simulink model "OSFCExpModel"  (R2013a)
settings: Solver=ode3  StartTime=0.0  StopTime=10  FixedStep=Ts  RelTol=1e-3
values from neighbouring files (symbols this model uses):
  k1 = K(1)    [OSFC_Constants.m]
  k2 = K(2)    [OSFC_Constants.m]
  k3 = K(3)    [OSFC_Constants.m]
  k4 = K(4)    [OSFC_Constants.m]
  Rd = 0    [OSFC_Constants.m]
  Ri = 10    [OSFC_Constants.m]
  Ts = 0.01    [OSFC_Constants.m]
libraries: arduinolib x3, THLlib x2, simulink x2

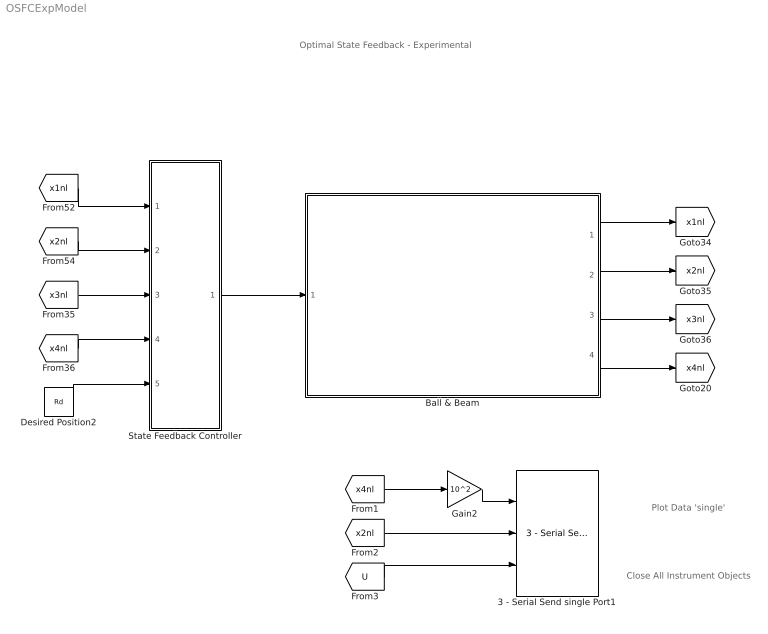
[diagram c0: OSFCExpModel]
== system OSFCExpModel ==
  note: Plot Data 'single'
  note: Close All Instrument Objects
  note: Optimal State Feedback - Experimental
  3 - Serial Send single Port1 : THLlib/3 - Serial Send  single Port0
  Ball & Beam : Subsystem
  Desired Position2 : Constant  Value=Rd
  Gain2 : Gain  Gain=10^2  SampleTime=Ts
  State Feedback Controller : Subsystem
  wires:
  [x1nl] -> State Feedback Controller/1(x1)
  [x2nl] -> State Feedback Controller/2(x2)
  [x3nl] -> State Feedback Controller/3(x3)
  [x4nl] -> State Feedback Controller/4(x4)
  Desired Position2/1 -> State Feedback Controller/5(R (desired))
  State Feedback Controller/1(U) -> Ball & Beam/1("U ")
  Ball & Beam/1(x1) -> [x1nl]
  Ball & Beam/2(x2) -> [x2nl]
  Ball & Beam/3(x3) -> [x3nl]
  Ball & Beam/4(x4) -> [x4nl]
  [x4nl] -> Gain2/1
  Gain2/1 -> 3 - Serial Send single Port1/1
  [x2nl] -> 3 - Serial Send single Port1/2
  [U] -> 3 - Serial Send single Port1/3

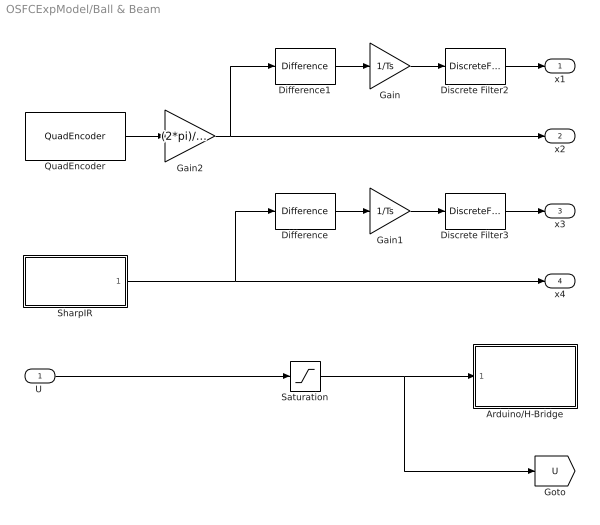
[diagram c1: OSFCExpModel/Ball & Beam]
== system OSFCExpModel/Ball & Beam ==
  "U " : Inport
  Arduino/H-Bridge : Subsystem
  Difference : simulink/Discrete/Difference  ICPrevInput=0.0  InputProcessing=Inherited  OutMin=[]  OutMax=[]  OutDataType=fixdt(1, 16)  OutScaling=2^-10  DoSatur=off
  Difference1 : simulink/Discrete/Difference  ICPrevInput=0.0  InputProcessing=Inherited  OutMin=[]  OutMax=[]  OutDataType=fixdt(1, 16)  OutScaling=2^-10  DoSatur=off
  Discrete Filter2 : DiscreteFilter  Numerator=[.4]  Denominator=[1 -0.6]  SampleTime=Ts
  Discrete Filter3 : DiscreteFilter  Numerator=[.4]  Denominator=[1 -0.6]  SampleTime=Ts
  Gain : Gain  Gain=1/Ts  SampleTime=Ts
  Gain1 : Gain  Gain=1/Ts  SampleTime=Ts
  Gain2 : Gain  Gain=(2*pi)/1336  SampleTime=Ts
  QuadEncoder : THLlib/QuadEncoder
  Saturation : Saturate  UpperLimit=12  LowerLimit=-12  SampleTime=Ts
  SharpIR : Subsystem
  x1 : Outport
  x2 : Outport  Port=2
  x3 : Outport  Port=3
  x4 : Outport  Port=4
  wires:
  "U "/1 -> Saturation/1
  Saturation/1 -> [U], Arduino/H-Bridge/1(ControlInput)
  Gain/1 -> Discrete Filter2/1
  Gain1/1 -> Discrete Filter3/1
  Difference1/1 -> Gain/1
  Difference/1 -> Gain1/1
  Discrete Filter3/1 -> x3/1
  Discrete Filter2/1 -> x1/1
  SharpIR/1(Out1) -> Difference/1, x4/1
  QuadEncoder/1 -> Gain2/1
  Gain2/1 -> x2/1, Difference1/1

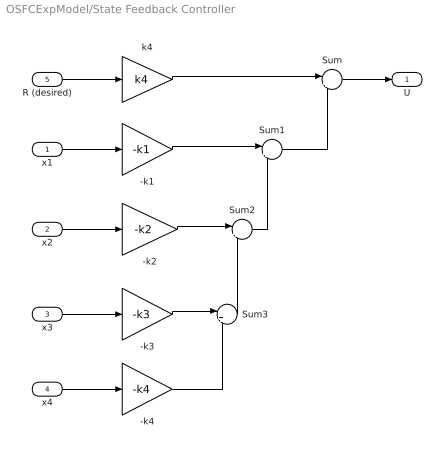
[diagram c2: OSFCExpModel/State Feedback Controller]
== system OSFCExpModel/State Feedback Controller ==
  x1 : Inport
  x2 : Inport  Port=2
  x3 : Inport  Port=3
  x4 : Inport  Port=4
  R (desired) : Inport  Port=5
  -k1 : Gain  Gain=-k1
  -k2 : Gain  Gain=-k2
  -k3 : Gain  Gain=-k3
  -k4 : Gain  Gain=-k4
  Sum{,1..3} (4 alike) : Sum  Inputs=|++
  k4 : Gain  Gain=k4
  U : Outport
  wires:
  -k4/1 -> Sum3/2
  Sum3/1 -> Sum2/2
  Sum2/1 -> Sum1/2
  Sum1/1 -> Sum/2
  Sum/1 -> U/1
  -k3/1 -> Sum3/1
  -k2/1 -> Sum2/1
  -k1/1 -> Sum1/1
  k4/1 -> Sum/1
  x4/1 -> -k4/1
  x3/1 -> -k3/1
  x2/1 -> -k2/1
  x1/1 -> -k1/1
  R (desired)/1 -> k4/1

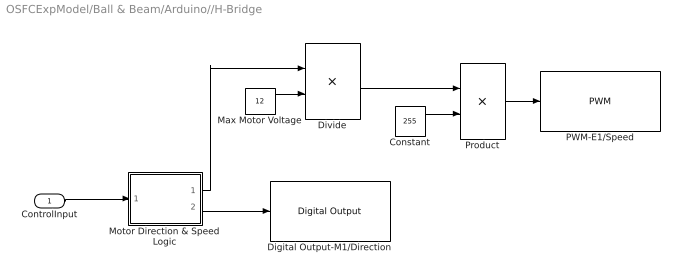
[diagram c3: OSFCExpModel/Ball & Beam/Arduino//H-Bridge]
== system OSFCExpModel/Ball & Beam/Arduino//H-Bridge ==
  ControlInput : Inport
  Constant : Constant  Value=255
  Digital Output-M1/Direction : arduinolib/Digital Output  pinNumber=4
  Divide : Product  Inputs=*/
  Max Motor Voltage : Constant  Value=12
  Motor Direction & Speed Logic : MATLAB Function  TreatAsAtomicUnit=on
  PWM-E1/Speed : arduinolib/PWM  pinNumber=5
  Product : Product
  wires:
  ControlInput/1 -> Motor Direction & Speed Logic/1(x)
  Constant/1 -> Product/2
  Product/1 -> PWM-E1/Speed/1
  Max Motor Voltage/1 -> Divide/2
  Divide/1 -> Product/1
  Motor Direction & Speed Logic/1(y) -> Divide/1
  Motor Direction & Speed Logic/2(y1) -> Digital Output-M1/Direction/1

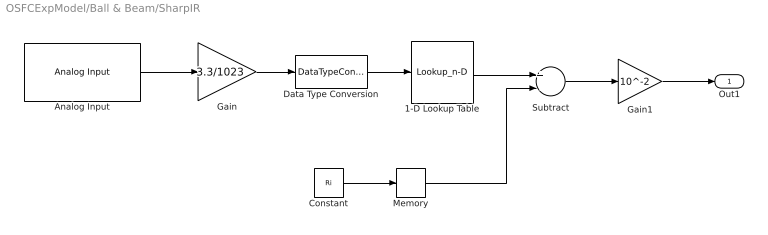
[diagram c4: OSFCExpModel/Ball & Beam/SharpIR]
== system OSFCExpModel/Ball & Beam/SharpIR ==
  1-D Lookup Table : Lookup_n-D  NumberOfTableDimensions=1  BreakpointsForDimension1=[0.3000 0.3750 0.4250 0.5200 0.6300 0.7250 0.8150 0.9250 1.0700 1.2500 1.4000 1.5750 1.7750 2.0200 2.3500 2.7150 3.0000 3.0250]  BreakpointsForDimension1DataTypeStr=single  Table=[40 35 30 25 20 18 16 14 12 10 9 8 7 6 5 4 3.5 3]  TableDataTypeStr=single  IntermediateResultsDataTypeStr=single  OutDataTypeStr=single  RndMeth=Simplest  FractionDataTypeStr=single
  Analog Input : arduinolib/Analog Input  pinNumber=0  sampleTime=Ts
  Constant : Constant  Value=Ri  SampleTime=Ts
  Data Type Conversion : DataTypeConversion  OutDataTypeStr=single
  Gain : Gain  Gain=3.3/1023
  Gain1 : Gain  Gain=10^-2  SampleTime=Ts
  Memory : Memory
  Subtract : Sum  Inputs=+-  SampleTime=Ts
  Out1 : Outport
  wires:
  Gain1/1 -> Out1/1
  Constant/1 -> Memory/1
  Memory/1 -> Subtract/2
  1-D Lookup Table/1 -> Subtract/1
  Subtract/1 -> Gain1/1
  Data Type Conversion/1 -> 1-D Lookup Table/1
  Gain/1 -> Data Type Conversion/1
  Analog Input/1 -> Gain/1
